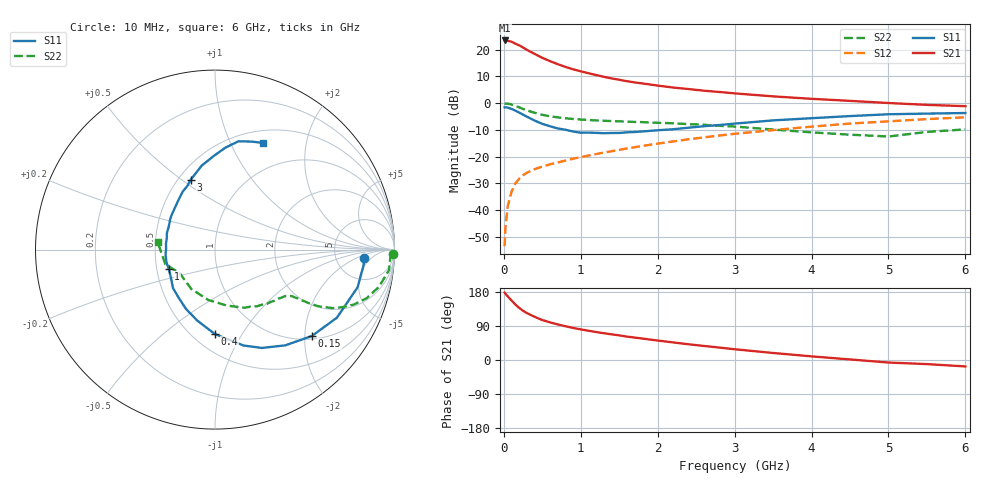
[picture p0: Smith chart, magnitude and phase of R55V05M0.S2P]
! SIEMENS Small Signal Semiconductors
! BFR183
! Si NPN RF Bipolar Junction Transistor in SOT23
! VCE = 5 V  IC = 5 mA
! Common Emitter S-Parameters:  May  1996
# GHz  S  MA  R  50
!  f  S11  S21  S12  S22
! GHz  MAG  ANG  MAG  ANG  MAG  ANG  MAG  ANG
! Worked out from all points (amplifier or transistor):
!   36 points, 10 MHz to 6 GHz, reference 50 ohm
!   highest |S21| = 23.4 dB at 10 MHz (marker M1)
!   |S21| within 3 dB of that: start of sweep to 270.5 MHz
!   unconditionally stable (mu >= 1): 1.053 GHz to 2.669 GHz
!   at 250 MHz: K = 0.42, MSG = 23.9 dB, |S12| = -27.0 dB
!   at 1.4 GHz: K = 1.06, MAG = 12.1 dB, |S12| = -18.0 dB
!   at 6 GHz: K = 0.88, MSG = 2.1 dB, |S12| = -5.3 dB
!   lowest NFmin = 1.15 dB at 450 MHz
!   S11 on the Smith chart (normalised r, x): 10 MHz: 10, -3; 150 MHz: 1.08, -2.17; 400 MHz: 0.64, -0.77; 1 GHz: 0.58, -0.13; 3 GHz: 0.58, +0.54; 6 GHz: 0.64, +1.33
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0.01  0.8326 -3.1  14.84 177.6  0.0021 88.0  0.9901 -1.3
0.02  0.8326 -6.0  14.67 174.9  0.0046 89.1  0.9776 -2.7
0.05  0.8218 -14.8  14.6 168.1  0.0116 81.6  0.9763 -6.7
0.1  0.7778 -29.2  14.06 157.0  0.022 75.5  0.9367 -12.8
0.15  0.7234 -41.7  12.92 146.3  0.0313 69.8  0.8869 -17.8
0.2  0.6619 -53.7  12.03 137.5  0.0384 65.5  0.8318 -21.6
0.25  0.6071 -64.5  10.96 129.8  0.0447 61.8  0.7751 -24.5
0.3  0.5572 -73.5  9.897 123.8  0.0497 59.6  0.7306 -26.5
0.4  0.4705 -90.1  8.311 114.0  0.058 56.5  0.6578 -28.7
0.5  0.4077 -104.0  7.019 105.5  0.0646 56.0  0.6023 -29.7
0.6  0.3681 -116.0  6.085 99.3  0.0714 55.8  0.5651 -30.2
0.8  0.3173 -137.6  4.749 89.1  0.0839 56.5  0.5193 -30.9
1  0.2788 -157.5  3.924 80.8  0.0971 57.5  0.4915 -31.7
1.1  0.2798 -165.1  3.618 77.3  0.1043 58.3  0.4816 -32.5
1.3  0.2726 179.8  3.098 70.7  0.1187 58.7  0.4659 -34.0
1.6  0.2836 160.8  2.565 61.8  0.1415 58.9  0.4485 -37.3
2.2  0.3237 133.4  1.952 46.4  0.1914 57.2  0.4189 -46.1
3  0.4126 109.1  1.519 28.4  0.2659 51.2  0.3635 -63.0
3.5  0.4742 98.9  1.334 18.5  0.3121 45.9  0.3194 -77.8
4.5  0.5707 84.2  1.099 1.5  0.4135 34.2  0.256 -121.0
5.5  0.6354 71.3  0.925 -10.8  0.5012 21.9  0.2885 -163.5
6  0.6512 66.0  0.875 -17.0  0.5417 13.7  0.3216 172.8
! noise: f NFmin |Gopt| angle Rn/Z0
0.45  1.15  0.25  40  0.26
0.9  1.2  0.25  93  0.22
1.8  1.95  0.32  170  0.13
